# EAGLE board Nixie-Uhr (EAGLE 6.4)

No outline drawn. Coordinates in mm, seen from the top.
Copper layers (1*16): Top 0.035mm / dielectric 1.5mm / Bottom 0.035mm
Design rules "default": minimum track width 10mil, minimum drill 24mil, track to track 8mil, track to pad 8mil, pad to pad 8mil, via to via 8mil, smd to smd 8mil, copper to edge 40mil, drill to drill 8mil, minimum pad ring 10mil, minimum via ring 8mil, stop-mask expansion 4mil, vias tented up to drill 0mil, thermal gap 10mil
Holes 1 mm at -31.25,5 -31.25,-5 31.25,5 31.25,-5 -33.75,5 -28.75,5 -33.75,-5 -28.75,-5 28.75,5 33.75,5 28.75,-5 33.75,-5 -3.81,19.32 -1.27,19.32 3.81,19.32 -2.54,25.4 0,25.4 2.54,25.4 -62.5,31.25 -62.5,28.75 62.5,31.25 62.5,28.75
Holes 6.5 mm at 31.25,5 31.25,-5 -31.25,5 -31.25,-5

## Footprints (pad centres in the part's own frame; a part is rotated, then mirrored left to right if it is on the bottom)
IN-12 = hole 1: 0,9; 0,-9; 0,-9; -5.75,0; 5.75,0; -5.75,4.5; 5.75,4.5; 5.75,-4.5; -5.75,-4.5; -4,-8; 4,-8; 4,8; -4,8 | hole 4: 0,0

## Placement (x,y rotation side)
E$1  [IN-12]  -75,0 0 top
E$2  [IN-12]  -50,0 0 top
E$3  [IN-12]  -12.5,0 0 top
E$4  [IN-12]  12.5,0 0 top
E$5  [IN-12]  50,0 0 top
E$6  [IN-12]  75,0 0 top

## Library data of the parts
E$1-E$6 = Nixie_IN-12

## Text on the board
Reference: TSOP / 4838 | PFW351 | PFW351 | TSOP1738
